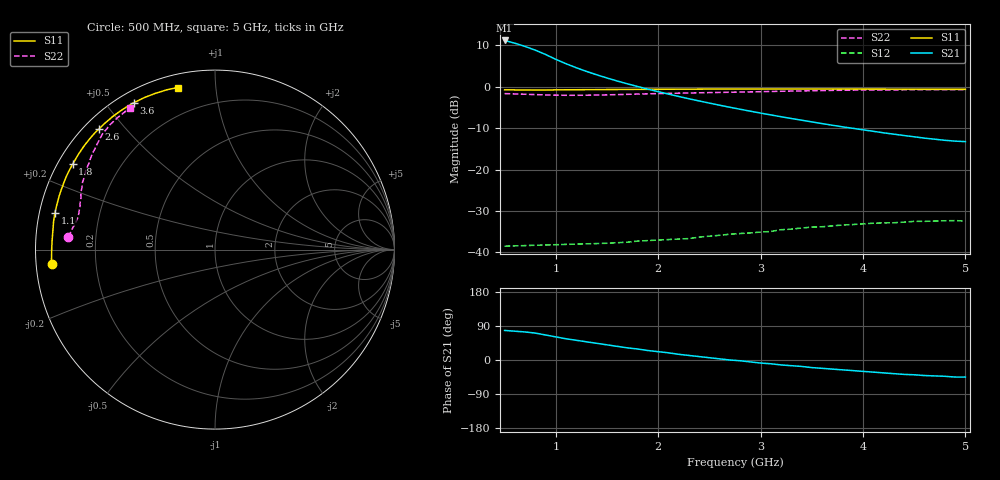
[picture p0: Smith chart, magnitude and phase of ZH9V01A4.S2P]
! SIEMENS Discrete & RF Semiconductors
! CLY38
! GaAs Power FET in MWP-35
! VDS = 9 V  ID = 1400 mA
! Common Source S-Parameters:  August  1998
# GHz  S  MA  R  50
!  f  S11  S21  S12  S22
! GHz  MAG  ANG  MAG  ANG  MAG  ANG  MAG  ANG
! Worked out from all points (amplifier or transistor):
!   46 points, 500 MHz to 5 GHz, reference 50 ohm
!   highest |S21| = 11.1 dB at 500 MHz (marker M1)
!   |S21| within 3 dB of that: start of sweep to 863.3 MHz
!   unconditionally stable (mu >= 1): 768.7 MHz to end of sweep
!   at 1.2 GHz: K = 1.53, MAG = 17.0 dB, |S12| = -38.0 dB
!   at 2.8 GHz: K = 2.00, MAG = 9.3 dB, |S12| = -35.4 dB
!   at 5 GHz: K = 2.22, MAG = 3.4 dB, |S12| = -32.4 dB
!   S11 on the Smith chart (normalised r, x): 500 MHz: 0.05, -0.04; 1.1 GHz: 0.04, +0.11; 1.8 GHz: 0.04, +0.28; 2.6 GHz: 0.04, +0.42; 3.6 GHz: 0.05, +0.59; 5 GHz: 0.06, +0.79
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0.5  0.914 -175.0  3.599 78.0  0.0119 17.0  0.823 175.0
0.7  0.91 180.0  3.048 74.0  0.0121 15.0  0.808 173.0
0.8  0.909 177.0  2.747 71.0  0.0122 15.0  0.801 171.0
0.9  0.909 174.0  2.439 66.0  0.0123 14.0  0.793 170.0
1  0.913 170.0  2.13 61.0  0.0124 13.0  0.788 168.0
1.1  0.915 167.0  1.886 56.0  0.0125 12.0  0.785 167.0
1.2  0.916 164.0  1.687 52.0  0.0126 12.0  0.785 165.0
1.3  0.918 161.0  1.523 48.0  0.0127 13.0  0.787 164.0
1.4  0.919 159.0  1.386 44.0  0.0128 13.0  0.79 162.0
1.6  0.923 154.0  1.167 36.0  0.0131 14.0  0.8 159.0
1.7  0.924 152.0  1.079 32.0  0.0133 15.0  0.806 158.0
1.8  0.925 149.0  1.001 29.0  0.0137 16.0  0.812 157.0
2  0.928 145.0  0.868 22.0  0.0141 16.0  0.823 154.0
2.2  0.93 142.0  0.76 15.0  0.0145 17.0  0.833 151.0
2.6  0.933 134.0  0.596 3.0  0.0161 17.0  0.85 146.0
2.8  0.934 131.0  0.533 -2.0  0.0169 17.0  0.859 144.0
3  0.935 128.0  0.479 -8.0  0.0176 17.0  0.868 142.0
3.5  0.935 120.0  0.375 -20.0  0.0202 17.0  0.891 136.0
3.6  0.935 119.0  0.358 -22.0  0.0204 16.0  0.895 135.0
4.3  0.931 110.0  0.267 -36.0  0.0228 12.0  0.913 127.0
4.8  0.927 104.0  0.225 -43.0  0.0241 8.0  0.918 123.0
5  0.926 103.0  0.217 -45.0  0.0239 6.0  0.92 121.0
